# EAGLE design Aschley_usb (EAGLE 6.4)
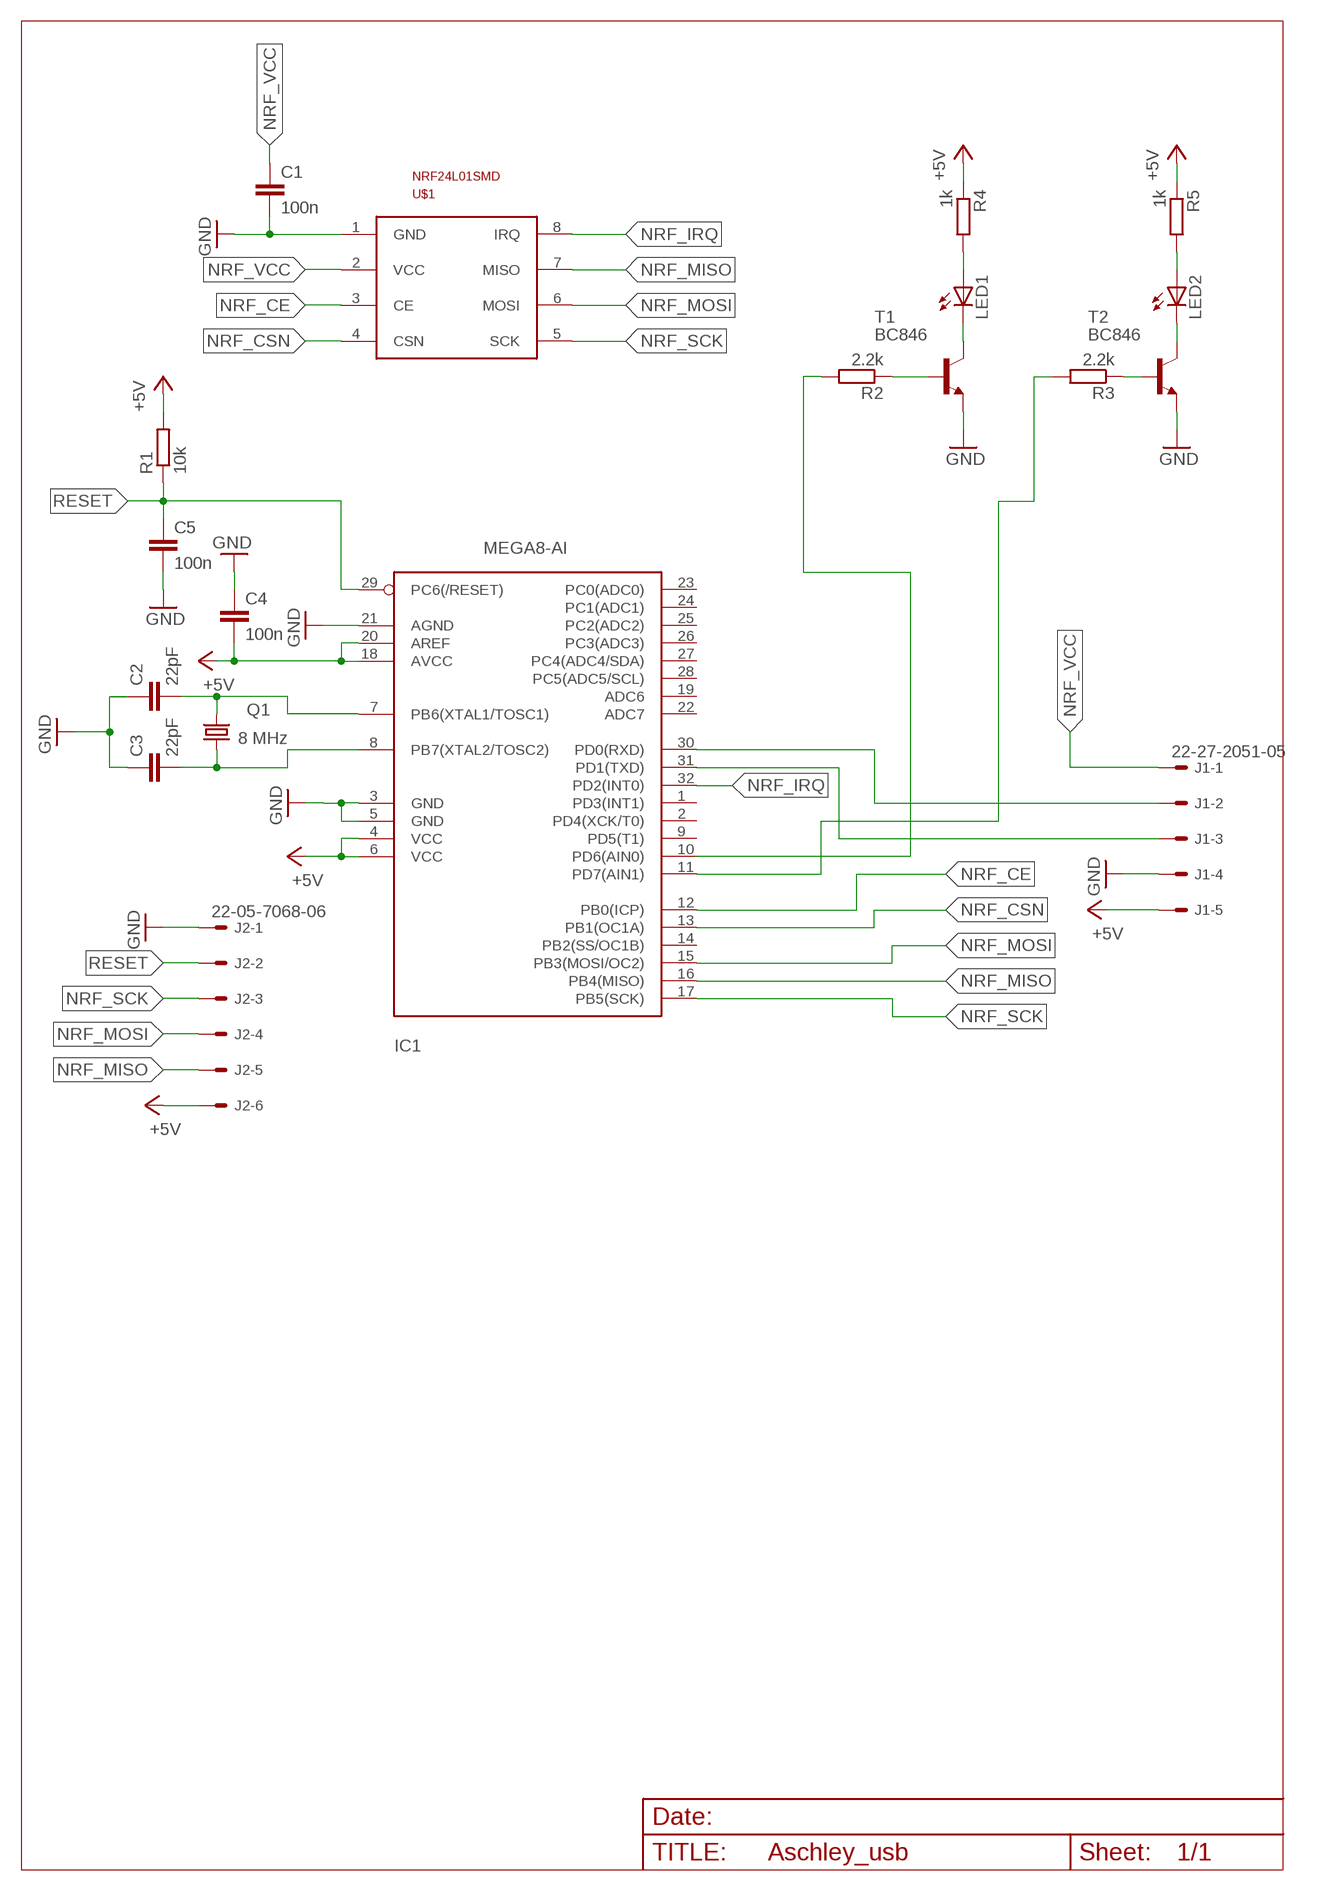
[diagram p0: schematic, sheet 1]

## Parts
C1  100n  C-EUC0805  [C0805]
C2  22pF  C-EUC0805  [C0805]
C3  22pF  C-EUC0805  [C0805]
C4  100n  C-EUC0805  [C0805]
C5  100n  C-EUC0805  [C0805]
IC1  MEGA8-AI  [TQFP32-08]
J1  22-27-2051-05  [6410-05]
J2  22-05-7068-06  [7395-06]
LED1  LEDSMT1206  [1206]
LED2  LEDSMT1206  [1206]
Q1  8 MHz  CRYSTALHC49S  [HC49/S]
R1  10k  R-EU_M0805  [M0805]
R2  2.2k  R-EU_M0805  [M0805]
R3  2.2k  R-EU_M0805  [M0805]
R4  1k  R-EU_M0805  [M0805]
R5  1k  R-EU_M0805  [M0805]
T1  BC846  [SOT23]
T2  BC846  [SOT23]
U$1  NRF24L01SMD  [NRF24L01SMD]

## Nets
+5V: C4.2 IC1.4(VCC) IC1.6(VCC) IC1.18(AVCC) IC1.20(AREF) J1.5 J2.6 R1.2 R4.1 R5.1
GND: C1.2 C2.1 C3.1 C4.1 C5.2 IC1.3(GND) IC1.5(GND) IC1.21(AGND) J1.4 J2.1 T1.2(E) T2.2(E) U$1.1(GND)
N$1: IC1.30(PD0(RXD)) J1.2
N$2: IC1.31(PD1(TXD)) J1.3
N$3: C3.2 IC1.8(PB7(XTAL2/TOSC2)) Q1.1
N$4: C2.2 IC1.7(PB6(XTAL1/TOSC1)) Q1.2
N$9: LED1.C T1.3(C)
N$10: LED2.C T2.3(C)
N$11: R2.1 T1.1(B)
N$12: R3.1 T2.1(B)
N$13: LED1.A R4.2
N$14: LED2.A R5.2
N$15: IC1.11(PD7(AIN1)) R3.2
N$16: IC1.10(PD6(AIN0)) R2.2
NRF_CE: IC1.12(PB0(ICP)) U$1.3(CE)
NRF_CSN: IC1.13(PB1(OC1A)) U$1.4(CSN)
NRF_IRQ: IC1.32(PD2(INT0)) U$1.8(IRQ)
NRF_MISO: IC1.16(PB4(MISO)) J2.5 U$1.7(MISO)
NRF_MOSI: IC1.15(PB3(MOSI/OC2)) J2.4 U$1.6(MOSI)
NRF_SCK: IC1.17(PB5(SCK)) J2.3 U$1.5(SCK)
NRF_VCC: C1.1 J1.1 U$1.2(VCC)
RESET: C5.1 IC1.29(PC6(/RESET)) J2.2 R1.1
Unconnected: IC1.1(PD3(INT1)) IC1.2(PD4(XCK/T0)) IC1.9(PD5(T1)) IC1.14(PB2(SS/OC1B)) IC1.19(ADC6) IC1.22(ADC7) IC1.23(PC0(ADC0)) IC1.24(PC1(ADC1)) IC1.25(PC2(ADC2)) IC1.26(PC3(ADC3)) IC1.27(PC4(ADC4/SDA)) IC1.28(PC5(ADC5/SCL))

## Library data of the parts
C1-C5 = rcl:C-EU: CAPACITOR, European symbol
IC1 = avr-7:MEGA8: MICROCONTROLLER 8 Kbytes FLASH 1 kbytes SRAM 512 bytes EEPROM USART 6-channel 10 bit ADC 2-channel 8 bit ADC
J1 = con-molex:22-?-05: CONNECTOR wire to board 2.54 mm (.1 inch) pitch header
J2 = con-molex:22-?-06: CONNECTOR wire to board 2.54 mm (.1 inch) pitch header
LED1 LED2 = ada:LED: LED
Q1 = ada:CRYSTAL: CRYSTAL; OC_FARNELL: 1667008; OC_NEWARK: unknown
R1-R5 = rcl:R-EU_: RESISTOR, European symbol
T1 T2 = transistor:BC846: NPN TRANSISTOR
U$1 = nrf24l01smd:NRF24L01SMD

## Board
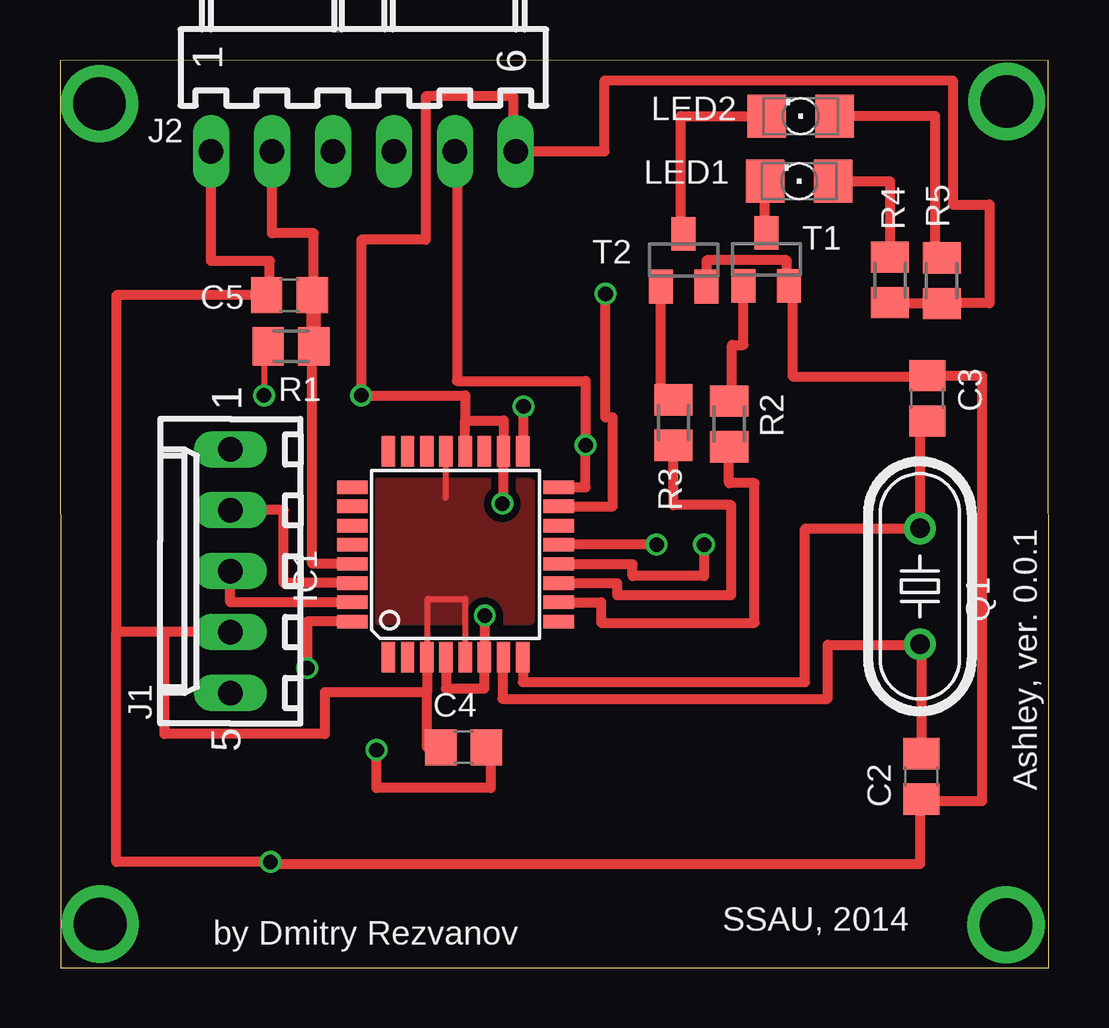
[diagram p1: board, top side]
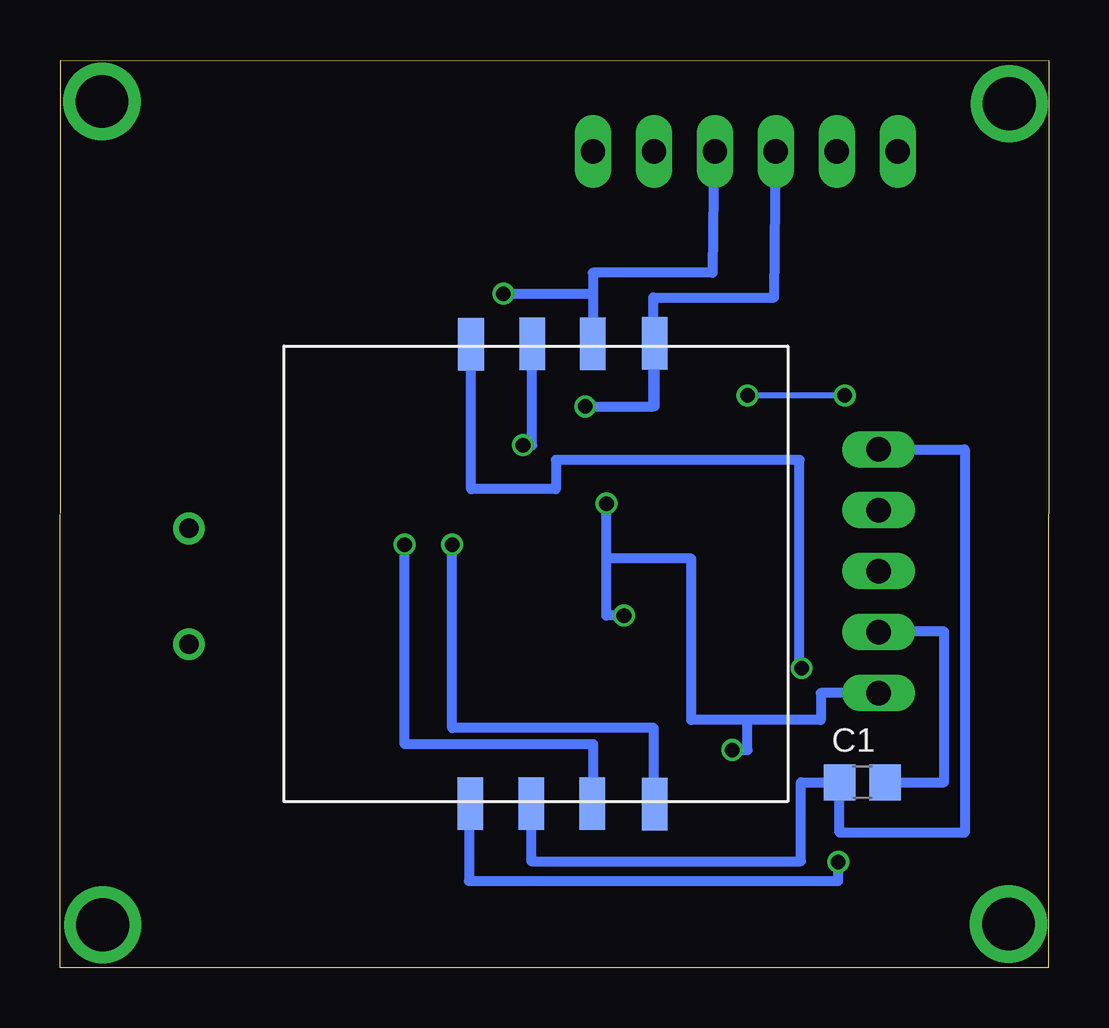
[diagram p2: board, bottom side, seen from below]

Size 41.22 x 37.85 mm. Coordinates in mm from the lower left corner, seen from the top.
Outline: 0.03,0 41.22,0 41.19,37.85 0,37.82 0.03,0
Copper layers (1*16): Top 0.035mm / dielectric 1.5mm / Bottom 0.035mm
Design rules "ITEADstudio_DRC": minimum track width 6mil, minimum drill 12mil, track to track 6mil, track to pad 6mil, pad to pad 6mil, via to via 6mil, smd to smd 0mil, copper to edge 10mil, drill to drill 10mil, minimum pad ring 10mil, minimum via ring 6mil, stop-mask expansion 2mil, vias tented up to drill 100mil, thermal gap 10mil

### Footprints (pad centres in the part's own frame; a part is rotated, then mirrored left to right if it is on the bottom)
C0805 = smd 1.3 x 1.5: 1 -0.95,0; 2 0.95,0
TQFP32-08 = smd 1.27 x 0.559: 1 -4.293,2.8; 2 -4.293,2; 3 -4.293,1.2; 4 -4.293,0.4; 5 -4.293,-0.4; 6 -4.293,-1.2; 7 -4.293,-2; 8 -4.293,-2.8; 17 4.293,-2.8; 18 4.293,-2; 19 4.293,-1.2; 20 4.293,-0.4; 21 4.293,0.4; 22 4.293,1.2; 23 4.293,2; 24 4.293,2.8 | smd 0.559 x 1.27: 9 -2.8,-4.293; 10 -2,-4.293; 11 -1.2,-4.293; 12 -0.4,-4.293; 13 0.4,-4.293; 14 1.2,-4.293; 15 2,-4.293; 16 2.8,-4.293; 25 2.8,4.293; 26 2,4.293; 27 1.2,4.293; 28 0.4,4.293; 29 -0.4,4.293; 30 -1.2,4.293; 31 -2,4.293; 32 -2.8,4.293
6410-05 = drill 1.016 long: 1 5.08,0; 2 2.54,0; 3 0,0; 4 -2.54,0; 5 -5.08,0
7395-06 = drill 1.016 long: 1 6.35,0; 2 3.81,0; 3 1.27,0; 4 -1.27,0; 5 -3.81,0; 6 -6.35,0
1206 = smd 1.6 x 1.803: A -1.422,0; C 1.422,0
HC49/S = drill 0.813: 1 -2.413,0; 2 2.413,0
M0805 = smd 1.3 x 1.6: 1 -0.95,0; 2 0.95,0
SOT23 = smd 1 x 1.4: 1 -0.95,-1.1; 2 0.95,-1.1; 3 0,1.1
NRF24L01SMD = smd 2.184 x 1.067: 1 0,0; 2 0,-2.54; 3 0,-5.08; 4 -0.022,-7.677; 5 19.172,-7.686; 6 19.167,-5.102; 7 19.151,-2.57; 8 19.142,-0.027

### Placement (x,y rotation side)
C1  7.77,7.74 0 bottom
C2  35.91,7.99 90 top
C3  36.15,23.74 270 top
C4  16.82,9.2 0 top
C5  9.57,28.04 180 top
IC1  16.49,17.24 90 top
J1  7.1,16.54 90 top
J2  12.65,34.05 180 top
LED1  30.82,32.8 180 top
LED2  30.88,35.51 180 top
Q1  35.84,15.91 270 top
R1  9.63,25.91 180 top
R2  27.89,22.68 270 top
R3  25.57,22.74 270 top
R4  34.59,28.68 90 top
R5  36.76,28.65 90 top
T1  29.44,29.54 0 top
T2  26,29.5 0 top
U$1  24.11,6.86 90 bottom

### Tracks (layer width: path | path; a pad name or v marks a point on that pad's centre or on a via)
+5V  (via drill 0.61)
  Top 0.254: IC1.20 | IC1.4 | R1.2 8.5,25.91 v8.5,23.87 | C4.2 17.69,9.2
  Top 0.406: IC1.20 16.89,22.83 | 16.89,22.83 18.49,22.83 IC1.18 18.49,19.35 v18.44,19.35 | v17.71,14.69 17.71,12.95 IC1.6 17.69,11.64 16.09,11.64 IC1.4 | 16.89,22.83 16.89,23.87 v12.56,23.87 12.56,30.36 15.24,30.36 15.24,36.33 18.9,36.33 18.9,34.05 J2.6 22.71,34.05 22.71,37 37.22,37 37.22,31.82 38.74,31.82 38.74,27.71 R5.1 34.6,27.7 R4.1 | 17.69,9.2 17.95,9.2 17.95,7.5 13.2,7.5 v13.2,9.08
  Bottom 0.254: v8.5,23.87 v12.56,23.87
  Bottom 0.406: v17.71,14.69 18.44,14.69 18.44,17.07 | 18.44,17.07 v18.44,19.35 | J1.5 9.51,11.46 9.51,10.33 12.56,10.33 | 12.56,10.33 14.91,10.33 14.91,17.07 18.44,17.07 | v13.2,9.08 12.56,9.08 12.56,10.33
GND  (via drill 0.61)
  Top 0.254: IC1.3 15.33,12.95 15.33,15.39 16.89,15.39 IC1.5 | IC1.21 16.06,21.53 16.06,19.6
  Top 0.406: IC1.3 15.3,12.95 15.3,11.49 | 15.3,11.49 11.03,11.49 11.03,9.75 4.36,9.75 4.36,14.02 | 4.36,14.02 7.1,14.02 J1.4 | 2.35,14.02 2.35,4.42 v8.78,4.42 8.78,4.33 35.84,4.33 35.84,6.95 35.91,6.95 | 2.35,14.02 4.36,14.02 | J2.1 6.3,29.47 8.75,29.47 8.75,28.04 C5.2 2.35,28.04 2.35,14.02 | C4.1 15.3,9.2 15.3,11.49 | C3.1 36.67,24.69 | 36.67,24.69 38.44,24.69 38.44,6.95 35.91,6.95 | 35.91,6.95 C2.1 | T2.2 26.95,29.5 30.3,29.5 30.3,28.43 T1.2 30.54,28.43 30.54,24.66 36.67,24.66 36.67,24.69
  Bottom 0.406: C1.2 4.36,7.74 4.36,14.02 7.1,14.02 J1.4 | U$1.1 24.17,6.86 24.17,3.63 8.78,3.63 v8.78,4.42
  pour Top (isolate 0.305): 13.23,14.51 19.6,14.51 19.6,20.21 13.23,20.21
N$1
  Top 0.406: IC1.30 9.33,16.04 9.33,19.08 J1.2 | J1.2
N$2
  Top 0.406: IC1.31 7.1,15.24 J1.3
N$3
  Top 0.406: IC1.8 19.29,11.92 31.06,11.92 31.06,18.32 Q1.1 35.84,22.79 C3.2
N$4
  Top 0.406: IC1.7 18.44,12.95 18.44,11.22 32,11.22 32,13.47 35.84,13.47 Q1.2 35.91,13.5 C2.2
N$5  (via drill 2.2)
  other vias: 1.65,36.03
N$6  (via drill 2.2)
  other vias: 39.47,36.12
N$7  (via drill 2.2)
  other vias: 39.44,1.8
N$8  (via drill 2.2)
  other vias: 1.68,1.83
N$9
  Top 0.406: T1.3 29.39,30.63 LED1.C
N$10
  Top 0.406: T2.3 25.88,30.6 25.88,35.51 LED2.C
N$11
  Top 0.406: R2.1 28.01,23.63 28.01,25.97 28.49,25.97 T1.1
N$12
  Top 0.406: R3.1 25.05,23.69 T2.1
N$13
  Top 0.406: LED1.A 34.6,32.8 R4.2
N$14
  Top 0.406: R5.2 36.48,29.6 36.48,35.51 LED2.A
N$15
  Top 0.406: IC1.11 23.23,16.04 23.23,15.54 27.98,15.54 27.98,19.29 25.57,19.29 R3.2
N$16
  Top 0.406: IC1.10 22.56,15.24 22.56,14.39 28.96,14.39 28.96,20.21 27.89,20.21 R2.2
NRF_CE  (via drill 0.61)
  Top 0.254: 20.78,16.82 IC1.12
  Top 0.406: v26.85,17.65 26.85,16.34 23.87,16.34 23.87,16.82 20.78,16.82
  Bottom 0.254: U$1.3 18.99,6.86
  Bottom 0.406: 18.99,6.86 18.99,9.33 26.85,9.33 v26.85,17.65
NRF_CSN  (via drill 0.61)
  Top 0.254: IC1.13
  Top 0.406: v24.87,17.65 IC1.13
  Bottom 0.254: U$1.4 16.46,6.84
  Bottom 0.406: 16.46,6.84 16.46,10 24.87,10 v24.87,17.65
NRF_IRQ  (via drill 0.61)
  Top 0.406: IC1.32 10.3,14.44 v10.3,12.5
  Bottom 0.406: v10.3,12.5 10.39,12.5 10.39,21.18 20.54,21.18 20.54,19.96 24.08,19.96 U$1.8
NRF_MISO  (via drill 0.61)
  Top 0.406: IC1.16 21.92,20.04 v21.92,21.79 21.92,24.48 16.55,24.48 16.55,34.05 J2.5
  Bottom 0.406: v21.92,21.79 21.54,21.79 U$1.7
NRF_MOSI  (via drill 0.61)
  Top 0.406: IC1.15 23.04,19.24 23.04,22.95 22.74,22.95 v22.74,28.1
  Bottom 0.406: v22.74,28.1 19.01,28.1 | 19.01,28.1 U$1.6 | J2.4 13.96,34.05 14.02,28.99 19.01,28.99 19.01,28.1
NRF_SCK  (via drill 0.61)
  Top 0.406: IC1.17 19.32,21.53 v19.32,23.41
  Bottom 0.406: v19.32,23.41 16.49,23.41 | U$1.5 16.42,23.41 16.49,23.41 | 16.49,23.41 16.49,27.95 11.44,27.95 J2.3
NRF_VCC
  Bottom 0.406: U$1.2 21.58,6.86 21.58,4.45 10.33,4.45 10.33,7.74 C1.1 | J1.1 3.51,21.62 3.51,5.64 8.72,5.64 C1.1 | C1.1
RESET
  Top 0.406: IC1.29 10.52,16.84 10.52,25.91 R1.1 | C5.1 10.58,28.04 10.58,30.63 8.84,30.63 J2.2
  Top 0.61: C5.1 10.58,28.04 R1.1

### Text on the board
tNames: Ashley, ver. 0.0.1 | by Dmitry Rezvanov | SSAU, 2014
